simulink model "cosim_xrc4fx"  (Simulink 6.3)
settings: Solver=ode45  StartTime=0.0  StopTime=10.0  RelTol=1e-3
undefined symbols (not defined in the file or in its folder): netlist_xrc4fx
libraries: xbsIndex_r4 x8, adlibrary2 x1, adcosim_example_lib x1

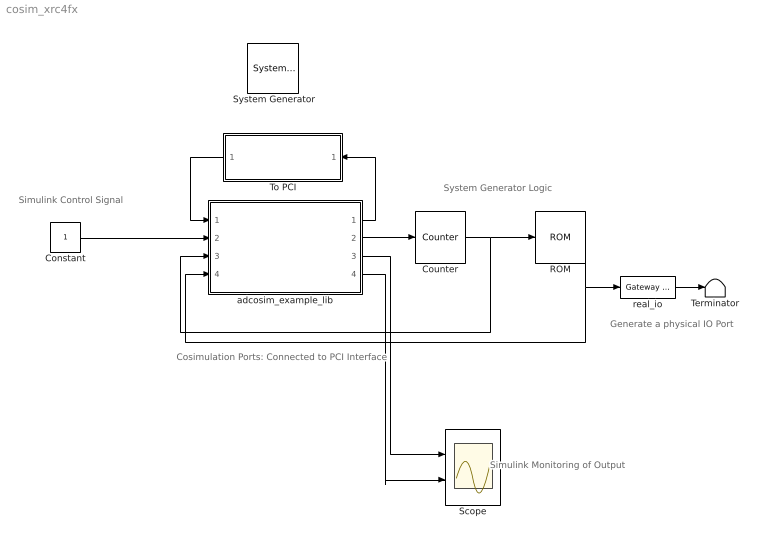
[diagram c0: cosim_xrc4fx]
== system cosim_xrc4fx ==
  note: System Generator Logic
  note: Simulink Control Signal
  note: Simulink Monitoring of Output
  note: Generate a physical IO Port
  note: Cosimulation Ports: Connected to PCI Interface
  " System Generator" : xbsIndex_r4/ System Generator  Tag=genX  xilinxfamily=Virtex4  part=xc4vfx100  speed=-10  package=ff1517  synthesis_tool=XST  directory=./netlist_xrc4fx  testbench=off  simulink_period=1  sysclk_period=6  incr_netlist=off  trim_vbits=Everywhere in SubSystem  dbl_ovrd=According to Block Masks  core_generation=According to Block Masks  run_coregen=off  deprecated_control=off  eval_field=0  block_type=sysgen
  Constant : Constant
  Counter : xbsIndex_r4/Counter  cnt_type=Free Running  cnt_to=Inf  operation=Up  start_count=0  cnt_by_val=1  arith_type=Unsigned  n_bits=8  bin_pt=0  load_pin=off  rst=off  en=on  dbl_ovrd=off  explicit_period=on  period=1  use_behavioral_HDL=off  use_rpm=off  block_type=counter
  ROM : xbsIndex_r4/ROM  depth=256  initVector=32767*sin(2*pi*(0:255)/256)  distributed_mem=Block RAM  rst=off  init_reg=0  en=off  latency=1  arith_type="Signed  (2's comp)"  n_bits=16  bin_pt=0  dbl_ovrd=off  use_rpm=on  block_type=sprom
  Scope : Scope  NumInputPorts=2
  Terminator : Terminator
  To PCI : Subsystem  Orientation=left
  adcosim_example_lib : Subsystem  Tag=configX  BlockChoice=adcosim_example_lib_sim
  real_io : xbsIndex_r4/Gateway Out  hdl_port=on  timing_constraint=None  locs_specified=on  LOCs={'H27','H28','N22','N23','J27','K27','C32','D32','H29','H30','J29','J30','E32','E33','P22','R21'}  block_type=gatewayout
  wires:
  Counter/1 -> ROM/1, adcosim_example_lib/3(count_sg)
  adcosim_example_lib/1(debug_out) -> To PCI/1(debug_out)
  To PCI/1(debug_in) -> adcosim_example_lib/1(debug_in)
  adcosim_example_lib/2(enable_sg) -> Counter/1
  ROM/1 -> adcosim_example_lib/4(sine_sg), real_io/1
  Constant/1 -> adcosim_example_lib/2(enable_sl)
  adcosim_example_lib/3(count_sl) -> Scope/1
  adcosim_example_lib/4(sine_sl) -> Scope/2
  real_io/1 -> Terminator/1

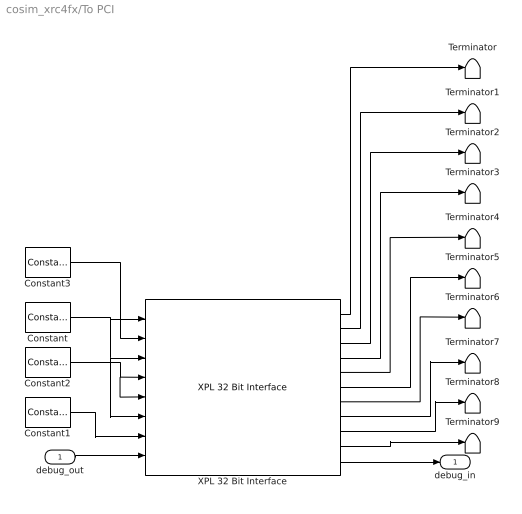
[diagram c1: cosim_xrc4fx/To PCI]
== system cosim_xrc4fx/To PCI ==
  debug_out : Inport
  Constant : xbsIndex_r4/Constant  arith_type=Unsigned  const=0  n_bits=32  bin_pt=0  explicit_period=on  period=1  equ=P=C  opselect=C  inp2=PCIN>>17  opr=+  inp1=P  carry=CIN  dbl_ovrd=off  block_type=constant
  Constant1 : xbsIndex_r4/Constant  arith_type=Unsigned  const=0  n_bits=66  bin_pt=0  explicit_period=on  period=1  equ=P=C  opselect=C  inp2=PCIN>>17  opr=+  inp1=P  carry=CIN  dbl_ovrd=off  block_type=constant
  Constant2 : xbsIndex_r4/Constant  arith_type=Boolean  const=0  n_bits=1  bin_pt=0  explicit_period=on  period=1  equ=P=C  opselect=C  inp2=PCIN>>17  opr=+  inp1=P  carry=CIN  dbl_ovrd=off  block_type=constant
  Constant3 : xbsIndex_r4/Constant  arith_type=Boolean  const=1  n_bits=1  bin_pt=0  explicit_period=on  period=1  equ=P=C  opselect=C  inp2=PCIN>>17  opr=+  inp1=P  carry=CIN  dbl_ovrd=off  block_type=constant
  Terminator{,1..9} (10 alike) : Terminator
  XPL 32 Bit Interface : adlibrary2/ADM-XPL/XPL 32 Bit Interface  program=''  clock_ratio=1.5  sstep_clk_sel_default=0
  debug_in : Outport
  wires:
  XPL 32 Bit Interface/11 -> debug_in/1
  debug_out/1 -> XPL 32 Bit Interface/8
  XPL 32 Bit Interface/10 -> Terminator9/1
  XPL 32 Bit Interface/9 -> Terminator8/1
  XPL 32 Bit Interface/8 -> Terminator7/1
  XPL 32 Bit Interface/7 -> Terminator6/1
  XPL 32 Bit Interface/6 -> Terminator5/1
  XPL 32 Bit Interface/5 -> Terminator4/1
  XPL 32 Bit Interface/4 -> Terminator3/1
  XPL 32 Bit Interface/3 -> Terminator2/1
  XPL 32 Bit Interface/2 -> Terminator1/1
  XPL 32 Bit Interface/1 -> Terminator/1
  Constant/1 -> XPL 32 Bit Interface/3, XPL 32 Bit Interface/6, XPL 32 Bit Interface/1
  Constant1/1 -> XPL 32 Bit Interface/7
  Constant2/1 -> XPL 32 Bit Interface/5, XPL 32 Bit Interface/4
  Constant3/1 -> XPL 32 Bit Interface/2

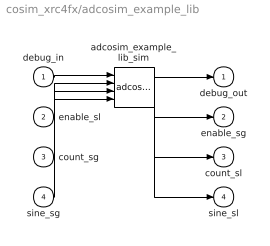
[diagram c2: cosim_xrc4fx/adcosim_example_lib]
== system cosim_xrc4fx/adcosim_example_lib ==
  debug_in : Inport
  enable_sl : Inport  Port=2
  count_sg : Inport  Port=3
  sine_sg : Inport  Port=4
  adcosim_example_lib_sim : adcosim_example_lib/adcosim_example_lib_sim
  debug_out : Outport
  enable_sg : Outport  Port=2
  count_sl : Outport  Port=3
  sine_sl : Outport  Port=4
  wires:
  debug_in/1 -> adcosim_example_lib_sim/1
  enable_sl/1 -> adcosim_example_lib_sim/2
  count_sg/1 -> adcosim_example_lib_sim/3
  sine_sg/1 -> adcosim_example_lib_sim/4
  adcosim_example_lib_sim/1 -> debug_out/1
  adcosim_example_lib_sim/2 -> enable_sg/1
  adcosim_example_lib_sim/3 -> count_sl/1
  adcosim_example_lib_sim/4 -> sine_sl/1
